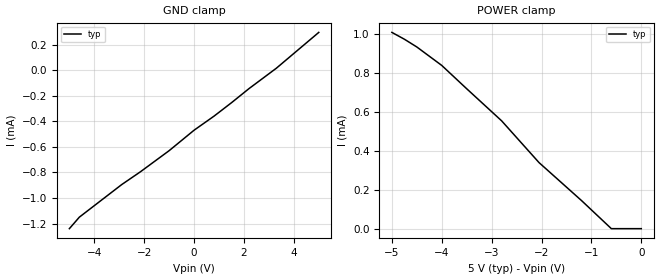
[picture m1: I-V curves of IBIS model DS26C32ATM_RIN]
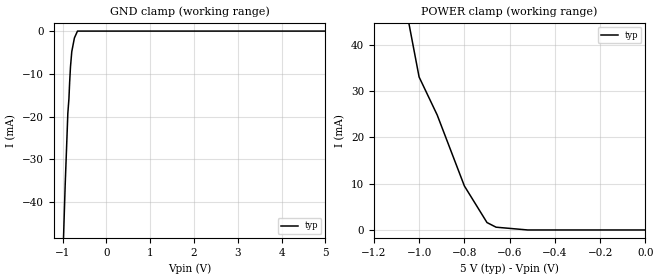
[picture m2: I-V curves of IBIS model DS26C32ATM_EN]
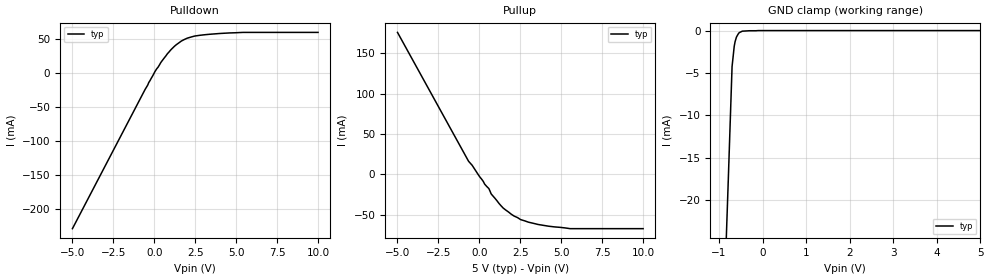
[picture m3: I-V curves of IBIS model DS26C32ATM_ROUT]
|   National Semiconductor Corporation
|   Interface Products Group
|   IBIS Model of DS26C32ATM
|   16L SOIC NARROW Package
[IBIS Ver]   3.2
[File name]   ds26c32atm.ibs
[File Rev]   1.1
[Date]   5/28/03
[Source]   File originated at National Semiconductor Corporation.
   Data Transmission Products group. All data based on
   Empirical Measurements(Bench).
[Notes]   All Data reused from the DS26C32 model;
   Only the pin parasitics modified;
   File created by Davor Glisic.
[Disclaimer]
(C) Copyright National Semiconductor Corporation 1994
   All rights reserved
   National Semiconductor Corporation hereby grants
the user of this IBIS model a non-exclusive, nontransferable
license to use this IBIS model under the following terms.
Before using this IBIS model, the user should read this
license.  If the user does not accept these terms,  the
IBIS model should be returned to National within 30 days.
   The user is granted this license only to use the
IBIS model and is not granted rights to sell, load, rent,
lease or license the IBIS model in whole or in part, or in
modified form to anyone other than user. User may modify
the IBIS model to suit its specific applications but rights
to derivative works and such modifications shall belong to
National.
   This IBIS model is provided on an "AS IS" basis and
National makes absolutely no warranty with respect to the
information contained herein.NATIONAL DISCLAIMS AND CUSTOMER
WAIVES ALL WARRANTIES, EXPRESS OR IMPLIED, INCLUDING
WARRANTIES OF MERCHANTABILITY OR FITNESS FOR A PARTICULAR
PURPOSE. The entire risk as to quality and performance is
with the Customer. ACCORDINGLY, IN NO EVENT SHALL THE
COMPANY BE LIABLE FOR ANY DAMAGES, WHETHER IN CONTRACT OR
TORT,INCLUDING ANY LOST PROFITS OR OTHER INCIDENTAL,
CONSEQUENTIAL, EXEMPLARY, OR PUNITIVE DAMAGES ARISING OUT
OF THE USE OR APPLICATION OF THE IBIS model provided in
this package.Further, National reserves the right to make
changes without notice to any product herein to improve
reliability, function, or design. National does not convey
any license under patent rights or any other intellectual
property rights, including those of third parties.
   National is not obligated to provide maintenance or support
for the licensed IBIS model.
Contact National at ATTN:INTERFACE APPLICATIONS/IBIS MODELS.
2900 Semiconductor Drive, M/S A2595, Santa Clara, CA 95052-8090
[Disclaimer] IBIS Open Forum disclaims all warranties. See DISCLAIM.TXT
   in vhdl.org:/pub/IBIS/models for the full disclaimer.
[Copyright]   Copyright 1994, National Semiconductor, All Rights Reserved
[Component]   DS26C32ATM
[Manufacturer]  National Semiconductor Corp
[Package]
|   typ   min   max
R_pkg   50.0m   50.0m   50.0m
L_pkg   1.37nH   0.95nH   2.07nH
C_pkg   0.26pF   0.152pF   0.429pF
[Pin]   signal_name   model_name   R_pin   L_pin   C_pin
1   RINA-   DS26C32ATM_RIN   50.0m   2.07nH   0.429pF
2   RINA+   DS26C32ATM_RIN   50.0m   1.49nH   0.306pF
3   ROUTA   DS26C32ATM_ROUT   50.0m   0.95nH   0.146pF
4   EN   DS26C32ATM_EN   50.0m   0.95nH   0.152pF
5   ROUTC   DS26C32ATM_ROUT   50.0m   0.95nH   0.152pF
6   RINC+   DS26C32ATM_RIN   50.0m   0.95nH   0.146pF
7   RINC-   DS26C32ATM_RIN   50.0m   1.49nH   0.306pF
8   GND   GND   50.0m   2.07nH   0.429pF
9   RIND-   DS26C32ATM_RIN   50.0m   2.07nH   0.429pF
10   RIND+   DS26C32ATM_RIN   50.0m   2.07nH   0.306pF
11   ROUTD   DS26C32ATM_ROUT   50.0m   0.95nH   0.146pF
12   EN*   DS26C32ATM_EN   50.0m   0.95nH   0.152pF
13   ROUTB   DS26C32ATM_ROUT   50.0m   0.95nH   0.152pF
14   RINB+   DS26C32ATM_RIN   50.0m   0.95nH   0.146pF
15   RINB-   DS26C32ATM_RIN   50.0m   1.49nH   0.306pF
16   VCC   POWER   50.0m   2.07nH   0.429pF
[Diff_pin]   inv_pin   vdiff   tdelay_typ   tdelay_min   tdelay_max
| The '+' pin is Diff_pin and the '-' pin is the inv_pin
2   1   0.2   0 0 0  | Receiver Vth=+/-200mV
6   7   0.2   0 0 0
10   9   0.2   0 0 0
14   15   0.2   0 0 0
| Models and submodels in the file (3): DS26C32ATM_RIN (Input), DS26C32ATM_EN (Input), DS26C32ATM_ROUT (3-state)
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|   Receiver Input  MODEL
[Model]   DS26C32ATM_RIN
Model_type   Input
|Signals   RINA-,RINA+,RINC+,RINC-,RIND-,RIND+,RINB+,RINB-
Vinh = 2.0
Vinl = 0.8
|   typ   min   max
C_comp   1.0pF   NA   NA
|   typ   min   max
[Temperature Range]   25.0   NA   NA
[Voltage range]   5.0V   4.5V   5.5V
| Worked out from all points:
|   POWER clamp passes 1 mA (typ) near -4.93 V on its own axis
[Power_clamp]
| Note that the[POWER_clamp]voltage table is referenced to Vcc
| and is calculated using Vtable=Vcc - Vmeasured.
|   Voltage   I(typ)   I(min)   I(max)
-5V       1.01mA     NA         NA
-4.75V    975uA      NA         NA
-4.5V     935uA      NA         NA
-4V       840uA      NA         NA
-3.5V     720uA      NA         NA
-2.8V     555uA      NA         NA
-2.05V    340uA      NA         NA
-1.2V     145uA      NA         NA
-600mV    0A         NA         NA
0V        0A         NA         NA
[GND_clamp]
|   Voltage   I(typ)   I(min)   I(max)
-5V       -1.24mA    NA         NA
-4.6V     -1.15mA    NA         NA
-3.6V     -1mA       NA         NA
-2.9V     -895uA     NA         NA
-2.15V    -795uA     NA         NA
-1V       -630uA     NA         NA
0V        -470uA     NA         NA
800mV     -360uA     NA         NA
1.5V      -255uA     NA         NA
2.2V      -145uA     NA         NA
3.3V      15uA       NA         NA
5V        295uA      NA         NA
|   Receiver Enable  MODEL
[Model]   DS26C32ATM_EN
Model_type   Input
|Signals   EN,EN*
Vinh = 2.0
Vinl = 0.8
|   typ   min   max
C_comp   1.0pF   NA   NA
|   typ   min   max
[Temperature Range]   25.0   NA   NA
[Voltage range]   5.0V   4.5V   5.5V
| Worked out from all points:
|   GND clamp passes 1 mA (typ) near -0.70 V on its own axis
|   POWER clamp passes 1 mA (typ) near -0.68 V on its own axis
[GND_clamp]
|   Voltage   I(typ)   I(min)   I(max)
-5V       -1.26A     NA         NA
-1.05V    -71.6mA    NA         NA
-940mV    -35.8mA    NA         NA
-880mV    -19.2mA    NA         NA
-855mV    -15.8mA    NA         NA
-840mV    -12.2mA    NA         NA
-820mV    -8.4mA     NA         NA
-790mV    -4.8mA     NA         NA
-730mV    -1.6mA     NA         NA
-660mV    0A         NA         NA
5V        0A         NA         NA
[Power_clamp]
| Note that the[POWER_clamp]voltage table is referenced to Vcc
| and is calculated using Vtable=Vcc - Vmeasured.
|   Voltage   I(typ)   I(min)   I(max)
-5V       1.06A      NA         NA
-1.06V    48.4mA     NA         NA
-1V       33mA       NA         NA
-920mV    24.8mA     NA         NA
-800mV    9.5mA      NA         NA
-700mV    1.6mA      NA         NA
-660mV    600uA      NA         NA
-520mV    0A         NA         NA
0V        0A         NA         NA
|   Receiver Output  MODEL
[Model]   DS26C32ATM_ROUT
Model_type   3-state
| Signals   ROUTA,ROUTB,ROUTC,ROUTD
Vmeas = 1.3V   |Reference voltage is at 50% of output swing
Cref = 50pF   |Timing specification test load capacitance value
Vref = 0   |Timing specification test load voltage; GND
| variable   typ   min   max
C_comp   3.0pF   NA   NA
|   typ   min   max
[Temperature Range]   25.0   NA   NA
[Voltage range]   5.0V   4.5V   5.5V
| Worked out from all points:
|   slope of the pulldown table from 0 to 0.75 V, typ, clamps not added: 28.4 ohm
|   slope of the pullup table from 0 to 0.75 V, typ, clamps not added: 33.3 ohm
|   GND clamp passes 1 mA (typ) near -0.61 V on its own axis
[Pulldown]
|   Voltage   I(typ)   I(min)   I(max)
-5V       -229.4mA   NA         NA
-560mV    -24.6mA    NA         NA
40mV      1.6mA      NA         NA
400mV     15mA       NA         NA
800mV     27.8mA     NA         NA
1.36V     41.4mA     NA         NA
1.66V     46.6mA     NA         NA
2V        50.6mA     NA         NA
2.46V     53.8mA     NA         NA
3.36V     56.4mA     NA         NA
5.42V     59.2mA     NA         NA
10V       59.2mA     NA         NA
[Pullup]
|   Voltage   I(typ)   I(min)   I(max)
| Note that the[Pullup]voltage table is referenced to Vcc
| and is calculated using Vtable=Vcc - Vmeasured.
-5V       175.6mA    NA         NA
-660mV    16.2mA     NA         NA
-440mV    11.2mA     NA         NA
320mV     -12mA      NA         NA
580mV     -17.6mA    NA         NA
720mV     -24.2mA    NA         NA
1.46V     -41.8mA    NA         NA
1.94V     -49.2mA    NA         NA
2.52V     -56mA      NA         NA
4.24V     -64.2mA    NA         NA
5.54V     -67.2mA    NA         NA
10V       -67.2mA    NA         NA
[GND_clamp]
|   Voltage   I(typ)   I(min)   I(max)
| Outputs in Tri-state.
-5V       -649.2mA   NA         NA
-790mV    -18.15mA   NA         NA
-700mV    -4.25mA    NA         NA
-650mV    -1.83mA    NA         NA
-630mV    -1.29mA    NA         NA
-600mV    -770uA     NA         NA
-560mV    -400uA     NA         NA
-535mV    -230uA     NA         NA
-465mV    -60uA      NA         NA
5V        10uA       NA         NA
[POWER_clamp]
|   Voltage   I(typ)   I(min)   I(max)
| Note that the[POWER_clamp]voltage table is referenced to Vcc
| and is calculated using Vtable=Vcc - Vmeasured.
| Outputs in Tri-state.
-5V       0A         NA         NA
0V        0A         NA         NA
4V        0A         NA         NA
5V        0A         NA         NA
[Ramp]
|   typ   min   max
dV/dt_r   2.8/1.3n   NA   NA
dV/dt_f   2.8/1.3n   NA   NA
R_load = 1MOhm
